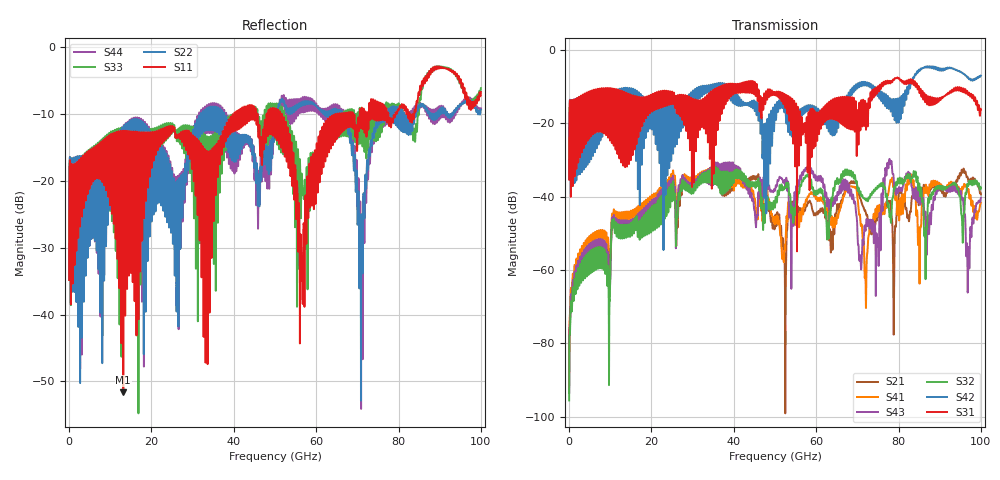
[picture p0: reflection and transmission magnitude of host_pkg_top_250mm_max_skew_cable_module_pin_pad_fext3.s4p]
# Hz S RI R 50
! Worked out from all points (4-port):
!   10000 points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, 10 MHz to 100 GHz, reference 50 ohm
!   strongest paths, dB at 10 MHz, 25.01 GHz, 50.01 GHz, 75.01 GHz, 100 GHz:
!     S31: -35.4, -11.4, -11.5, -10.0, -16.2
!     S42: -35.3, -14.4, -15.0, -11.9, -7.0
!     S32: -95.6, -41.3, -42.8, -37.3, -37.8
!     S43: -93.5, -39.0, -38.4, -52.7, -40.3
!     S41: -91.8, -37.3, -47.1, -44.3, -41.7
!     S21: -93.7, -39.0, -46.6, -45.1, -39.4
!   lowest |S11| = -51.6 dB at 13.16 GHz (marker M1), VSWR 1.01, Z = 49.8 + j0.184 ohm
!   |S11| at or under -10 dB: start of sweep to 40.15 GHz; 45.77 GHz to 47.96 GHz (2.195 GHz wide, 4.68 % of centre); 51.7 GHz to 64.72 GHz (13.02 GHz wide, 22.4 % of centre)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
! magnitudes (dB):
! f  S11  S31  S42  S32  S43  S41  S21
! 10 MHz  -34.8  -35.4  -35.3  -95.6  -93.5  -91.8  -93.7
! 13.16 GHz  -51.6  -25.5  -11.4  -47.7  -46.5  -44.2  -45.7
! 49.84 GHz  -9.1  -12.3  -19.3  -42.2  -38.2  -47.0  -48.7
! 56.44 GHz  -34.7  -18.7  -18.0  -36.4  -34.5  -44.9  -43.9
! 70.88 GHz  -11.9  -14.9  -9.9  -39.6  -59.8  -48.0  -41.0
! 77.78 GHz  -11.4  -8.5  -14.0  -45.4  -29.8  -37.1  -41.6
! 100 GHz  -6.7  -16.2  -7.0  -37.8  -40.3  -41.7  -39.4
